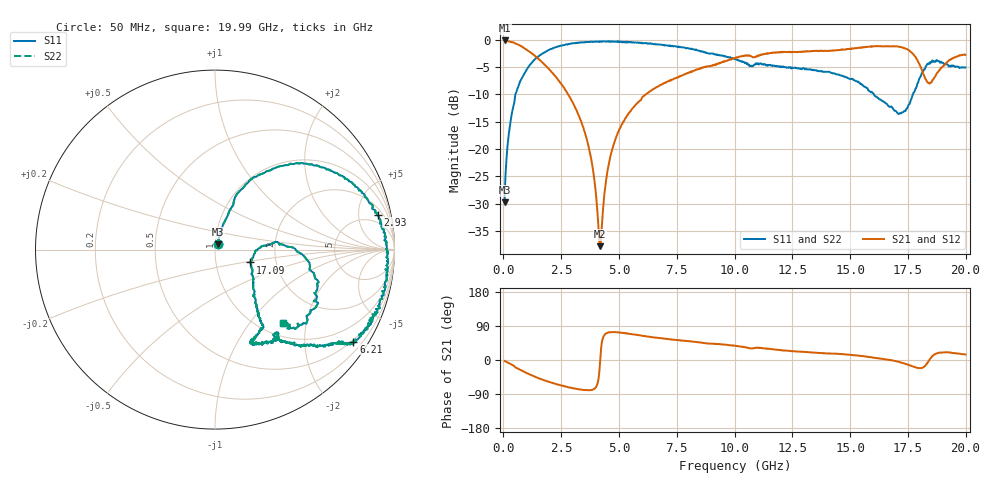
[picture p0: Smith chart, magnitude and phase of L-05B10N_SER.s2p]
! Data Taken on a HP 8720C VNA using a series-through fixture with TRL* de-embedding
#	mhz	s	ma	r	50
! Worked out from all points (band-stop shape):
!   998 points, 50 MHz to 19.99 GHz, reference 50 ohm
!   highest |S21| = -0.10 dB at 50 MHz (marker M1); lowest = -37.8 dB at 4.19 GHz (marker M2)
!   |S21| within 3 dB of the highest: start of sweep to 1.419 GHz; 10.91 GHz to 17.83 GHz (6.916 GHz wide, 48.1 % of centre)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
!   lowest |S11| = -29.8 dB at 50 MHz (marker M3), VSWR 1.07, Z = 51.4 + j3 ohm
!   |S11| at or under -10 dB: start of sweep to 516.6 MHz; 16.03 GHz to 17.71 GHz (1.68 GHz wide, 9.96 % of centre)
!   |S22| runs from -29.8 to -0.2 dB; largest |S21 - S12| = 0
!   S11 on the Smith chart (normalised r, x): 50 MHz: 1.03, +0.06; 2.93 GHz: 3.02, +8.32; 6.21 GHz: 0.45, -3.25; 17.09 GHz: 1.47, -0.22; 19.99 GHz: 1.25, -1.49
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50  0.03248 63.7  0.9882 -2.6  0.9882 -2.6  0.03248 63.7
310  0.1806 70.5  0.9597 -10.9  0.9597 -10.9  0.1806 70.5
750  0.4282 63.5  0.8766 -26.7  0.8766 -26.7  0.4282 63.5
1570  0.7216 40.7  0.6546 -49.4  0.6546 -49.4  0.7216 40.7
2930  0.9265 12.1  0.2834 -73.6  0.2834 -73.6  0.9265 12.1
3390  0.9475 4.5  0.1709 -78.6  0.1709 -78.6  0.9475 4.5
3830  0.9601 -1.8  0.07378 -78.8  0.07378 -78.8  0.9601 -1.8
4190  0.9677 -7.6  0.01288 3.5  0.01288 3.5  0.9677 -7.6
4490  0.9716 -12.3  0.06087 71.4  0.06087 71.4  0.9716 -12.3
4810  0.9626 -17.5  0.117 73.5  0.117 73.5  0.9626 -17.5
6210  0.926 -33.6  0.3213 62.0  0.3213 62.0  0.926 -33.6
6710  0.9076 -35.2  0.3771 58.3  0.3771 58.3  0.9076 -35.2
10030  0.6666 -51.2  0.6859 37.7  0.6859 37.7  0.6666 -51.2
12070  0.5618 -68.0  0.7682 25.4  0.7682 25.4  0.5618 -68.0
13350  0.5294 -64.3  0.788 19.4  0.788 19.4  0.5294 -64.3
15150  0.4324 -55.5  0.8331 12.5  0.8331 12.5  0.4324 -55.5
16670  0.2464 -33.7  0.8719 0.6  0.8719 0.6  0.2464 -33.7
17090  0.2096 -19.9  0.8678 -4.7  0.8678 -4.7  0.2096 -19.9
17890  0.3825 4.0  0.6627 -20.3  0.6627 -20.3  0.3825 4.0
18390  0.6057 -19.3  0.4029 -3.5  0.4029 -3.5  0.6057 -19.3
18930  0.6311 -42.3  0.5551 19.8  0.5551 19.8  0.6311 -42.3
19990  0.5594 -47.1  0.7307 14.5  0.7307 14.5  0.5594 -47.1
